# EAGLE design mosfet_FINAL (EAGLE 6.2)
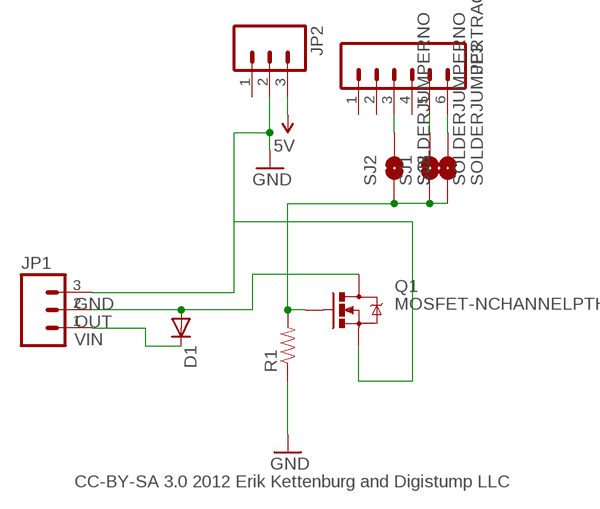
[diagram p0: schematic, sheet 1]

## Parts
D1  DIODEPTH  [DIODE-1N4001]
JP1  M03SCREW  [SCREWTERMINAL-3.5MM-3]
JP2  M03PTH  [1X03]
JP3  M06SIP  [1X06]
Q1  MOSFET-NCHANNELPTH2  [TO220V]
R1  RESISTORAXIAL-0.3  [AXIAL-0.3]
SJ1  SOLDERJUMPERNO  [SJ_2S-NO]
SJ2  SOLDERJUMPERNO  [SJ_2S-NO]
SJ3  SOLDERJUMPERTRACE  [SJ_2S-TRACE]

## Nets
5V: JP2.3
GND: JP1.3 JP2.2 Q1.3(S) R1.P$1
N$1: D1.A JP1.2 Q1.2(D)
N$3: D1.C JP1.1
N$4: JP3.6 SJ3.2
N$5: JP3.3 SJ2.2
N$6: Q1.1(G) R1.P$2 SJ1.1 SJ2.1 SJ3.1
N$7: JP3.5 SJ1.2
Unconnected: JP2.1 JP3.1 JP3.2 JP3.4

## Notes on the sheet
- GND
- OUT
- VIN
- CC-BY-SA 3.0 2012 Erik Kettenburg and Digistump LLC

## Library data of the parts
D1 = SparkFun:DIODE: Diode
JP1 JP2 = SparkFun:M03: Header 3 Standard 3-pin 0.1" header. Use with straight break away headers (SKU : PRT-00116), right angle break away headers (PRT-00553), swiss pins (PRT-00743), machine pins (PRT-00117), and female headers (PRT-00115). Molex polarized connector foot print use with SKU : PRT-08232 with associated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
JP3 = SparkFun:M06: Header 6 Standard 6-pin 0.1" header. Use with straight break away headers (SKU : PRT-00116), right angle break away headers (PRT-00553), swiss pins (PRT-00743), machine pins (PRT-00117), and female headers (PRT-00115). Molex polarized connector foot print use with SKU : PRT-08094 with associated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
Q1 = SparkFun:MOSFET-NCHANNEL
R1 = SparkFun:RESISTOR: Resistor
SJ1-SJ3 = SparkFun:SOLDERJUMPER: Solder Jumper

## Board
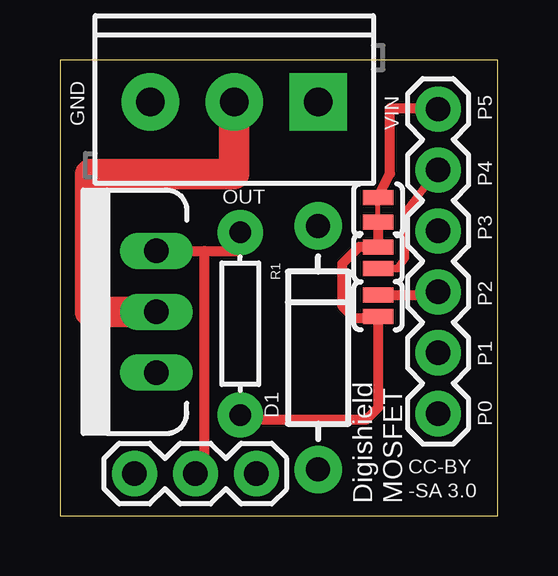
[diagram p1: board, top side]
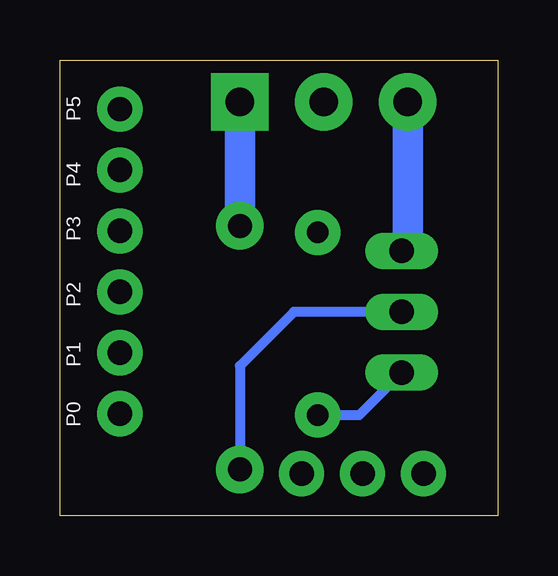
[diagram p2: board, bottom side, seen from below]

Size 18.25 x 19 mm. Coordinates in mm from the lower left corner, seen from the top.
Outline: 0,19 0,0 18.25,0 18.25,19 0,19
Copper layers (1*16): Top 0.0356mm / dielectric 1.5011mm / Bottom 0.0356mm
Design rules: minimum track width 8mil, minimum drill 13mil, track to track 10mil, track to pad 10mil, pad to pad 10mil, via to via 10mil, smd to smd 8mil, copper to edge 15mil, drill to drill 12mil, minimum pad ring 7mil, minimum via ring 7mil, stop-mask expansion 4mil, vias tented up to drill 24mil, thermal gap 10mil

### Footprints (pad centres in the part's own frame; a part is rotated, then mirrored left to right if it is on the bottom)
DIODE-1N4001 = drill 1 pad 1.981: A -5.08,0; C 5.08,0
SCREWTERMINAL-3.5MM-3 = drill 1.2 pad 2.413 square: 1 0,0 | drill 1.2 pad 2.413: 2 3.5,0; 3 7,0
1X03 = drill 1.016 pad 1.88: 1 0,0; 2 2.54,0; 3 5.08,0
1X06 = drill 1.016 pad 1.88: 1 0,0; 2 2.54,0; 3 5.08,0; 4 7.62,0; 5 10.16,0; 6 12.7,0
TO220V = drill 1.016 long: 1 -2.54,0; 2 0,0; 3 2.54,0
AXIAL-0.3 = drill 0.9 pad 1.88: P$1 -3.81,0; P$2 3.81,0
SJ_2S-NO = smd 0.635 x 1.27: 1 -0.45,0; 2 0.45,0
SJ_2S-TRACE = smd 0.635 x 1.27: 1 -0.508,0; 2 0.508,0

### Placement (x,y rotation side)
D1  10.75,7 90 top
JP1  10.75,17.25 180 top
JP2  8.17,1.75 180 top
JP3  15.75,4.25 90 top
Q1  4,8.5 90 top
R1  7.5,8 270 top
SJ1  13.25,10.75 270 top
SJ2  13.25,8.75 90 top
SJ3  13.25,12.75 90 top

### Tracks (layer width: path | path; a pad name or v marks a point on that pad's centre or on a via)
GND
  Top 0.406: R1.P$1 7.5,11.04 Q1.3 6,11.04 6,2 5.63,2 JP2.2
  Bottom 1.27: JP1.3 3.75,12.75 3.75,11.04 Q1.3
N$1
  Top 1.27: Q1.2 1.25,8.5 1.25,14.25 7.25,14.25 JP1.2
  Bottom 0.406: Q1.2 8.5,8.5 10.75,6.25 D1.A
N$3
  Bottom 1.27: D1.C JP1.1
N$4
  Top 0.406: SJ3.2 13.75,14.26 13.75,17 15.75,17 JP3.6
N$5
  Top 0.406: SJ2.2 15.62,9.2 JP3.3
N$6
  Top 0.406: SJ3.1 SJ1.1 12.45,11.2 11.75,10.5 11.75,8.75 12.25,8.25 13.2,8.25 SJ2.1 13.25,4.5 12.75,4 7.69,4 R1.P$2
  Bottom 0.406: R1.P$2 5.77,4.19 Q1.1
N$7
  Top 0.305: SJ1.2 14.05,10.3 14.38,10.75 14.38,12.66 JP3.5

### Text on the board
tPlace: VIN | GND | OUT | CC-BY | -SA 3.0 | Digishield | MOSFET
tNames: P5 | P4 | P3 | P2 | P1 | P0
bNames: P5 | P4 | P3 | P2 | P1 | P0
